(* Logix 5000 AddOnInstructionDefinition export B256_EtoDINT; software revision 30.00 *)

ADD_ON_INSTRUCTION D_SHL   (* revision 1.0, vendor Ken Fischer, NSWCPD, C512 *)
// DINT bit shift left of the 32-bit argument Inp_A by Inp_B bits with paddding by zeros on the right
// Revision note:
// Rev1.0: TBD - Initial Release
VAR_IN_OUT
   Inp_A : DINT; {required}   // 64-bit Integer to be right circular rotated
END_VAR
VAR_INPUT
   Inp_B : INT; {required}   // Number of bits to shift
END_VAR
VAR_IN_OUT
   Out : DINT; {required}   // Result
END_VAR
VAR
   Wrk_InpA : DINT[2];
   Source_Bit : BOOL;
   ONS : BOOL;
   BSL_Cntrl : CONTROL := (LEN := 32);
END_VAR

ROUTINE Logic   (* ladder *)
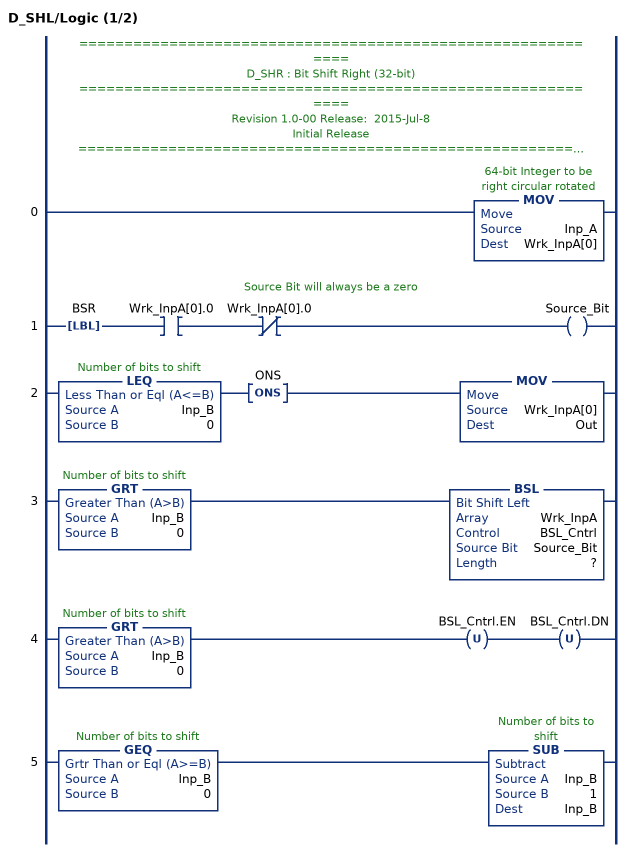
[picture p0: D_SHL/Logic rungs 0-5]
   // ============================================================
   // D_SHR : Bit Shift Right (32-bit)
   // ============================================================
   // Revision 1.0-00 Release:  2015-Jul-8
   // Initial Release
   // ============================================================
   // Performs a left bit shift of the 32-bit argument Inp_A by the
   // number of bits defined in the 16-bit argument Inp_B, with padding by zeros.
   0: MOV(Inp_A,Wrk_InpA[0]);
   // Source Bit will always be a zero
   1: LBL(BSR)XIC(Wrk_InpA[0].0)XIO(Wrk_InpA[0].0)OTE(Source_Bit);
   2: LEQ(Inp_B,0)ONS(ONS)MOV(Wrk_InpA[0],Out);
   3: GRT(Inp_B,0)BSL(Wrk_InpA,BSL_Cntrl,Source_Bit,?);
   4: GRT(Inp_B,0)OTU(BSL_Cntrl.EN)OTU(BSL_Cntrl.DN);
   5: GEQ(Inp_B,0)SUB(Inp_B,1,Inp_B);
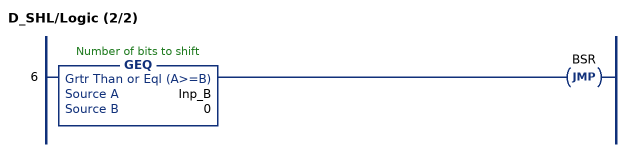
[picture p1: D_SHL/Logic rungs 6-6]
   6: GEQ(Inp_B,0)JMP(BSR);
END_ROUTINE
END_ADD_ON_INSTRUCTION

ADD_ON_INSTRUCTION B256_EtoDINT   (* revision 1.0 20170916, vendor Kenneth A. Fischer *)
// Convert 256-bit value using 32 8-bit pieces into 256-bit value using 8 32-bit pieces
// Revision note:
// Rev1.0: 20170916 - Initial Release
VAR_IN_OUT
   Inp_E : DINT[32]; {required}
   Out_DINT : DINT[8]; {required}
END_VAR
VAR
   D_SHL : D_SHL;
   i : INT;
   j : INT;
   TEMP : DINT;
END_VAR

ROUTINE Logic   (* ladder *)
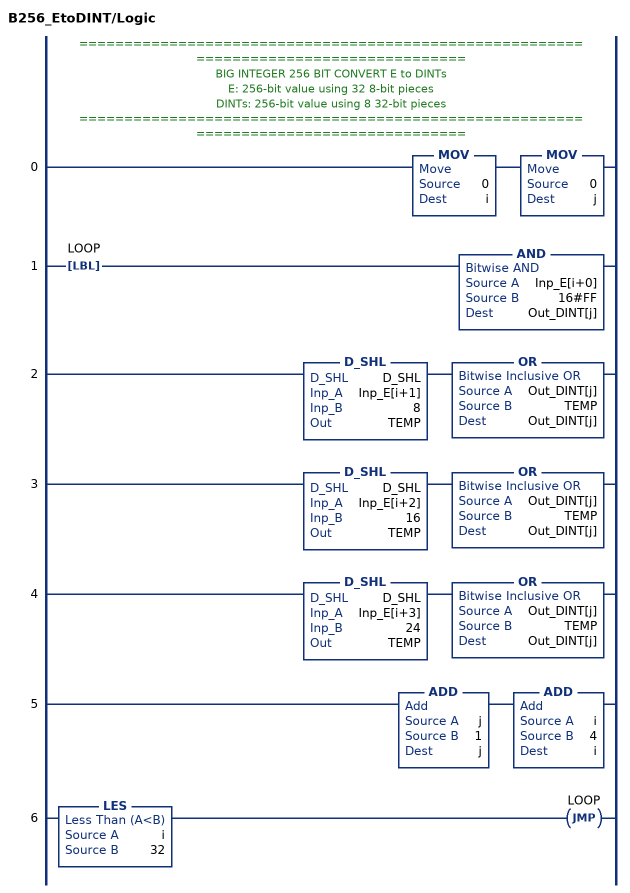
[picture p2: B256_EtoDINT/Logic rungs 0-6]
   // ======================================================================================
   // BIG INTEGER 256 BIT CONVERT E to DINTs
   // E: 256-bit value using 32 8-bit pieces
   // DINTs: 256-bit value using 8 32-bit pieces
   // ======================================================================================
   0: MOV(0,i)MOV(0,j);
   1: LBL(LOOP)AND(Inp_E[i+0],16#FF,Out_DINT[j]);
   2: D_SHL(D_SHL,Inp_E[i+1],8,TEMP)OR(Out_DINT[j],TEMP,Out_DINT[j]);
   3: D_SHL(D_SHL,Inp_E[i+2],16,TEMP)OR(Out_DINT[j],TEMP,Out_DINT[j]);
   4: D_SHL(D_SHL,Inp_E[i+3],24,TEMP)OR(Out_DINT[j],TEMP,Out_DINT[j]);
   5: ADD(j,1,j)ADD(i,4,i);
   6: LES(i,32)JMP(LOOP);
END_ROUTINE
END_ADD_ON_INSTRUCTION
